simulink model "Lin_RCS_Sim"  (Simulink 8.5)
settings: Solver=ode5  StartTime=0.0  StopTime=2500  FixedStep=Ts  MaxStep=0.005  RelTol=1e-3
InitFcn:
  | start
StartFcn:
  | start
StopFcn:
  | Pl
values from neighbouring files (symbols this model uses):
  Ave = [    [vehicle_flex34.m]    (also in vehicle_rigid.m)
  Bve = [    [vehicle_flex34.m]    (also in vehicle_rigid.m)
  Cve = [    [vehicle_flex34.m]    (also in vehicle_rigid.m)
  d2r = pi/180    (= 0.0174532925199)    [Dead_Band_DF.m]    (also in start.m; start1.m; start2.m; start3.m)
  Dve = [    [vehicle_flex34.m]    (also in vehicle_rigid.m)
  nt = 12    [start.m]    (also in start1.m; start2.m; start3.m)
  r2d = 180/pi    (= 57.2957795131)    [start.m]    (also in start1.m; start2.m; start3.m)
undefined symbols (not defined in the file or in its folder): Phase_Plane

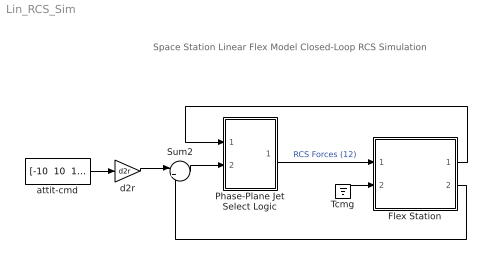
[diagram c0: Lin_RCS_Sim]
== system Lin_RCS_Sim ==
  note: Space Station Linear Flex Model Closed-Loop RCS Simulation
  Flex Station : Subsystem
  Phase-Plane Jet Select Logic : Subsystem
  Sum2 : Sum  Inputs=|+-
  Tcmg : Ground
  attit-cmd : Constant  Value="[-10  10  10]"
  d2r : Gain  Gain=d2r
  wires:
  Flex Station/1(wbf) -> Phase-Plane Jet Select Logic/1(rater)
  Phase-Plane Jet Select Logic/1(f(i)) -> Flex Station/1(Frcs)  "RCS Forces (12)"
  Sum2/1 -> Phase-Plane Jet Select Logic/2(atter)
  attit-cmd/1 -> d2r/1
  d2r/1 -> Sum2/1
  Flex Station/2(att) -> Sum2/2
  Tcmg/1 -> Flex Station/2(Tcmg)

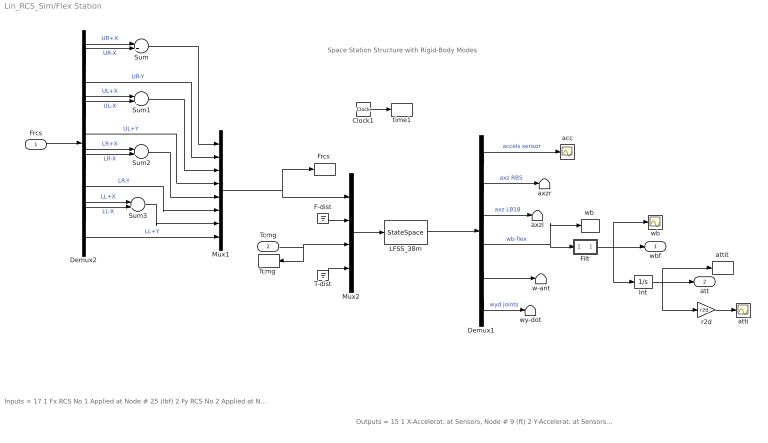
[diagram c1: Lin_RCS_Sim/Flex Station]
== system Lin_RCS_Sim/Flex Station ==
  note: Outputs = 15 1 X-Accelerat. at Sensors, Node # 9 (ft) 2 Y-Accelerat. at Sensors, Node # 9 (ft) 3 Z-Accelerat. at Sensors, Node # 9 (ft) 4 X-Accelerat. at Right Boom End, Node # 5 (ft) 5 Z-Accelerat. at Right Boom End, Node # 5 (ft) 6 X-Accelerat. at Left Boom End, Node # 18 (ft) 7 Z-Accelerat. at Left Boom End, Node # 18 (ft) 8 X-Rot. Rate at Sensors, Node # 9 (radian) 9 Y-Rot. Rate at Sensors, Node # 9 (radian) 10 Z-Rot. Rate at Sensors, Node # 9 (radian) 11 X-Rot. Rate at Antena Bot-Left, Node # 24 (radian) 12 Y-Rot. Rate at Antena Bot-Left, Node # 24 (radian) 13 Z-Rot. Rate at Antena Bot-Left, Node # 24 (radian) 14 Y-Rot.Accel. at Right Joint, Node # 7 (radian) 15 Y-Rot.Accel. at Left Joint, Node # 16 (radian)
  note: Inputs = 17 1 Fx RCS No 1 Applied at Node # 25 (lbf) 2 Fy RCS No 2 Applied at Node # 25 (lbf) 3 Fx RCS No 3 Applied at Node # 26 (lbf) 4 Fy RCS No 4 Applied at Node # 26 (lbf) 5 Fx RCS No 5 Applied at Node # 27 (lbf) 6 Fy RCS No 6 Applied at Node # 27 (lbf) 7 Fx RCS No 7 Applied at Node # 28 (lbf) 8 Fy RCS No 8 Applied at Node # 28 (lbf) 9 Fx Disturb. No 9 at Node # 21 (lbf) 10 Fy Disturb. No 10 at Node # 21 (lbf) 11 Fz Disturb. No 11 at Node # 21 (lbf) 12 Torq-x No 1 CMG Applied at Node # 10 (ft-lb) 13 Torq-y No 2 CMG Applied at Node # 10 (ft-lb) 14 Torq-z No 3 CMG Applied at Node # 10 (ft-lb) 15 Torq-x No 4 Gimbal Dist. at Node # 1 (ft-lb) 16 Torq-y No 5 Gimbal Dist. at Node # 1 (ft-lb) 17 Torq-z No 6 Gimbal Dist. at Node # 1 (ft-lb)
  note: Space Station Structure with Rigid-Body Modes
  Frcs : Inport
  Tcmg : Inport  Port=2
  Clock1 : Clock
  Demux1 : Demux  Outputs=[3, 2, 2, 3, 3, 2]
  Demux2 : Demux  Outputs=12
  F-dist : Ground
  Filt : Subsystem
  "Frcs " : ToWorkspace  VariableName=Frcs  SampleTime=-1
  Int : Integrator
  LFSS_38m : StateSpace  A=Ave  B=Bve  C=Cve  D=Dve  X0=0
  Mux1 : Mux  Inputs=8
  Mux2 : Mux  Inputs=[8, 3, 3, 3]
  Sum{,1..3} (4 alike) : Sum  Inputs=|+-
  T-dist : Ground
  "Tcmg " : ToWorkspace  VariableName=Tcmg  SampleTime=-1
  acc : Scope
  atti : Scope
  attit : ToWorkspace  VariableName=atti  SampleTime=-1
  axzl : Terminator
  axzr : Terminator
  r2d : Gain  Gain=r2d
  time1 : ToWorkspace  VariableName=time  SampleTime=-1
  w-ant : Terminator
  wb : Scope
  "wb " : ToWorkspace  VariableName=wb  SampleTime=-1
  wy-dot : Terminator
  wbf : Outport
  att : Outport  Port=2
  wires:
  Demux1/6 -> wy-dot/1  "wyd joints"
  Demux1/5 -> w-ant/1
  T-dist/1 -> Mux2/4
  F-dist/1 -> Mux2/2
  Demux1/3 -> axzl/1  "axz LB18"
  Demux1/2 -> axzr/1  "axz RB5"
  Tcmg/1 -> Mux2/3, "Tcmg "/1
  Demux1/4 -> "wb "/1, Filt/1(I)  "wb-flex"
  Demux1/1 -> acc/1  "accels sensor"
  LFSS_38m/1 -> Demux1/1
  Mux2/1 -> LFSS_38m/1
  Mux1/1 -> Mux2/1, "Frcs "/1
  Frcs/1 -> Demux2/1
  Demux2/6 -> Mux1/4  "UL+Y"
  Demux2/9 -> Mux1/6  "LR-Y"
  Demux2/12 -> Mux1/8  "LL+Y"
  Demux2/3 -> Mux1/2  "UR-Y"
  Demux2/1 -> Sum/1  "UR+X"
  Demux2/2 -> Sum/2  "UR-X"
  Sum/1 -> Mux1/1
  Demux2/4 -> Sum1/1  "UL+X"
  Demux2/5 -> Sum1/2  "UL-X"
  Sum1/1 -> Mux1/3
  Demux2/7 -> Sum2/1  "LR+X"
  Demux2/8 -> Sum2/2  "LR-X"
  Demux2/10 -> Sum3/1  "LL+X"
  Demux2/11 -> Sum3/2  "LL-X"
  Sum3/1 -> Mux1/7
  Sum2/1 -> Mux1/5
  r2d/1 -> atti/1
  Int/1 -> att/1, r2d/1, attit/1
  Clock1/1 -> time1/1
  Filt/1(O) -> wbf/1, Int/1, wb/1

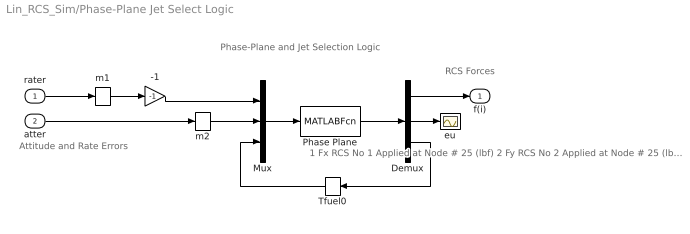
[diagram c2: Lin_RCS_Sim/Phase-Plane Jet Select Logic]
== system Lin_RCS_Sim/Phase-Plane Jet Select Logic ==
  note: Phase-Plane and Jet Selection Logic
  note: 1 Fx RCS No 1 Applied at Node # 25 (lbf) 2 Fy RCS No 2 Applied at Node # 25 (lbf) 3 Fx RCS No 3 Applied at Node # 26 (lbf) 4 Fy RCS No 4 Applied at Node # 26 (lbf) 5 Fx RCS No 5 Applied at Node # 27 (lbf) 6 Fy RCS No 6 Applied at Node # 27 (lbf) 7 Fx RCS No 7 Applied at Node # 28 (lbf) 8 Fy RCS No 8 Applied at Node # 28 (lbf)
  note: RCS Forces
  note: Attitude and Rate Errors
  rater : Inport
  atter : Inport  Port=2
  -1 : Gain  Gain=-1
  Demux : Demux  Outputs=[nt, 3,1]
  Mux : Mux  Inputs="[3  3  1]"
  Phase Plane : MATLABFcn  MATLABFcn=Phase_Plane( u(1:3), u(4:6), u(7) )  OutputDimensions=nt + 4
  Tfuel0 : Memory
  eu : Scope
  m1 : Memory
  m2 : Memory
  f(i) : Outport
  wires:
  Demux/3 -> Tfuel0/1
  -1/1 -> Mux/1
  atter/1 -> m2/1
  rater/1 -> m1/1
  Demux/2 -> eu/1
  Demux/1 -> f(i)/1
  Tfuel0/1 -> Mux/3
  Phase Plane/1 -> Demux/1
  Mux/1 -> Phase Plane/1
  m1/1 -> -1/1
  m2/1 -> Mux/2

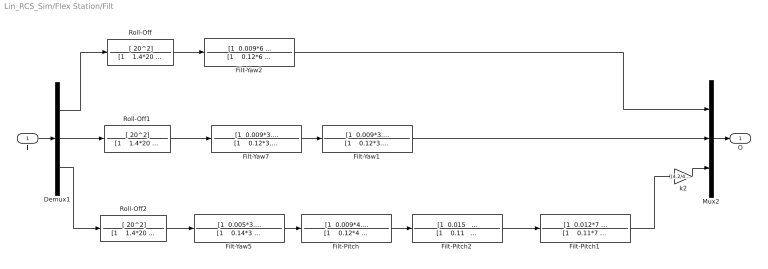
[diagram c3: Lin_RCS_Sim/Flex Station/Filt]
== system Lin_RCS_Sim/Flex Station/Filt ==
  I : Inport
  Demux1 : Demux  Outputs=3
  Filt-Pitch : TransferFcn  Numerator="[1  0.009*4.6   4.4^2]"  Denominator="[1    0.12*4    4.2^2]"
  Filt-Pitch1 : TransferFcn  Numerator="[1  0.012*7   6.85^2]"  Denominator="[1    0.11*7    6.85^2]"
  Filt-Pitch2 : TransferFcn  Numerator="[1  0.015   1.14^2]"  Denominator="[1    0.11    1.14^2]"
  Filt-Yaw1 : TransferFcn  Numerator="[1  0.009*3.9   3.93^2]"  Denominator="[1    0.12*3.9    3.93^2]"
  Filt-Yaw2 : TransferFcn  Numerator="[1  0.009*6   5.85^2]"  Denominator="[1    0.12*6    5.85^2]"
  Filt-Yaw5 : TransferFcn  Numerator="[1  0.005*3.1   3.09^2]"  Denominator="[1    0.14*3    3^2]"
  Filt-Yaw7 : TransferFcn  Numerator="[1  0.009*3.5   3.5^2]"  Denominator="[1    0.12*3.5    3.5^2]"
  Mux2 : Mux  Inputs=3
  Roll-Off : TransferFcn  Numerator=[ 20^2]  Denominator="[1    1.4*20    20^2]"
  Roll-Off1 : TransferFcn  Numerator=[ 20^2]  Denominator="[1    1.4*20    20^2]"
  Roll-Off2 : TransferFcn  Numerator=[ 20^2]  Denominator="[1    1.4*20    20^2]"
  k2 : Gain  Gain=(4.2/4.4)*(3/3.09)
  O : Outport
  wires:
  I/1 -> Demux1/1
  Mux2/1 -> O/1
  Demux1/1 -> Roll-Off/1
  Demux1/3 -> Roll-Off2/1
  Demux1/2 -> Roll-Off1/1
  Roll-Off/1 -> Filt-Yaw2/1
  Roll-Off2/1 -> Filt-Yaw5/1
  Roll-Off1/1 -> Filt-Yaw7/1
  Filt-Yaw5/1 -> Filt-Pitch/1
  Filt-Pitch/1 -> Filt-Pitch2/1
  k2/1 -> Mux2/3
  Filt-Yaw7/1 -> Filt-Yaw1/1
  Filt-Yaw1/1 -> Mux2/2
  Filt-Yaw2/1 -> Mux2/1
  Filt-Pitch1/1 -> k2/1
  Filt-Pitch2/1 -> Filt-Pitch1/1
